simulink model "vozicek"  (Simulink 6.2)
settings: Solver=ode45  StartTime=0.0  StopTime=100  RelTol=1e-3
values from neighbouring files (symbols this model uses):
  k1 = KK(1)    [ch8_d.m]    (also in set_x4a.m = 1; za_podmodel_voz.m = 1; auto_param.m = 7500; auto_param_opt.m = 15000)
  k2 = KK(2)    [ch8_d.m]    (also in set_x4a.m = 2; za_podmodel_voz.m = 2; auto_param.m = 150000; auto_param_opt.m = 150000)
  k3 = KK(3)    [ch8_d.m]    (also in set_x4a.m = 4; za_podmodel_voz.m = 4; INTEG_RK4.M = krm(2)*DERIV(t+0.5*krm(2),y+0.5*k2,par); kovinska_palica_2_RK4.m = 0.5)
  m1 = 10    [ex12_2st.m]    (also in set_x4a.m = 1; za_podmodel_voz.m = 1; Naloga31.m = 500)
  m2 = 5    [ex12_2st.m]    (also in set_x4a.m = 3; za_podmodel_voz.m = 3; Naloga31.m = 10)
  m3 = 2    [set_x4a.m]    (also in za_podmodel_voz.m)
  v10 = 0    [set_x4a.m]    (also in za_podmodel_voz.m)
  v20 = 0    [set_x4a.m]    (also in za_podmodel_voz.m)
  v30 = 0    [set_x4a.m]    (also in za_podmodel_voz.m)
  x10 = 1    [set_x4a.m]    (also in za_podmodel_voz.m)
  x20 = 0    [set_x4a.m]    (also in za_podmodel_voz.m)
  x30 = 0    [set_x4a.m]    (also in za_podmodel_voz.m)

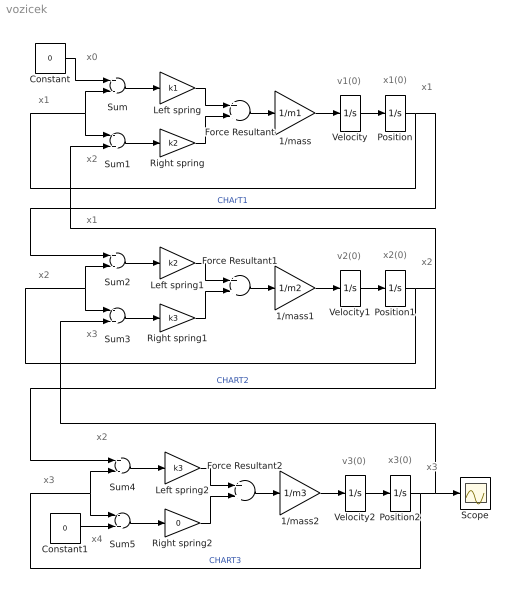
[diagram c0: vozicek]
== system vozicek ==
  note: x0
  note: x1
  note: x1
  note: x2
  note: v1(0)
  note: x1(0)
  note: x1
  note: x2
  note: x2
  note: x3
  note: v2(0)
  note: x2(0)
  note: x2
  note: x3
  note: x3
  note: x4
  note: v3(0)
  note: x3(0)
  1/mass : Gain  Gain=1/m1
  1/mass1 : Gain  Gain=1/m2
  1/mass2 : Gain  Gain=1/m3
  Constant : Constant  Value=0
  Constant1 : Constant  Value=0
  Force Resultant : Sum
  Force Resultant1 : Sum
  Force Resultant2 : Sum
  Left spring : Gain  Gain=k1
  Left spring1 : Gain  Gain=k2
  Left spring2 : Gain  Gain=k3
  Position : Integrator  InitialCondition=x10
  Position1 : Integrator  InitialCondition=x20
  Position2 : Integrator  InitialCondition=x30
  Right spring : Gain  Gain=k2
  Right spring1 : Gain  Gain=k3
  Right spring2 : Gain  Gain=0
  Scope : Scope
  Sum : Sum  Inputs=+-
  Sum1 : Sum  Inputs=-+
  Sum2 : Sum  Inputs=+-
  Sum3 : Sum  Inputs=-+
  Sum4 : Sum  Inputs=+-
  Sum5 : Sum  Inputs=-+
  Velocity : Integrator  InitialCondition=v10
  Velocity1 : Integrator  InitialCondition=v20
  Velocity2 : Integrator  InitialCondition=v30
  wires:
  Position/1 -> Sum1/1, Sum/2, Sum2/1  "CHArT1"
  Velocity/1 -> Position/1
  1/mass/1 -> Velocity/1
  Force Resultant/1 -> 1/mass/1
  Right spring/1 -> Force Resultant/2
  Left spring/1 -> Force Resultant/1
  Sum/1 -> Left spring/1
  Sum1/1 -> Right spring/1
  Constant/1 -> Sum/1
  Position1/1 -> Sum3/1, Sum2/2, Sum4/1, Sum1/2  "CHART2"
  Velocity1/1 -> Position1/1
  1/mass1/1 -> Velocity1/1
  Force Resultant1/1 -> 1/mass1/1
  Right spring1/1 -> Force Resultant1/2
  Left spring1/1 -> Force Resultant1/1
  Sum2/1 -> Left spring1/1
  Sum3/1 -> Right spring1/1
  Position2/1 -> Sum5/1, Sum4/2, Sum3/2, Scope/1  "CHART3"
  Velocity2/1 -> Position2/1
  1/mass2/1 -> Velocity2/1
  Force Resultant2/1 -> 1/mass2/1
  Right spring2/1 -> Force Resultant2/2
  Left spring2/1 -> Force Resultant2/1
  Sum4/1 -> Left spring2/1
  Sum5/1 -> Right spring2/1
  Constant1/1 -> Sum5/2
